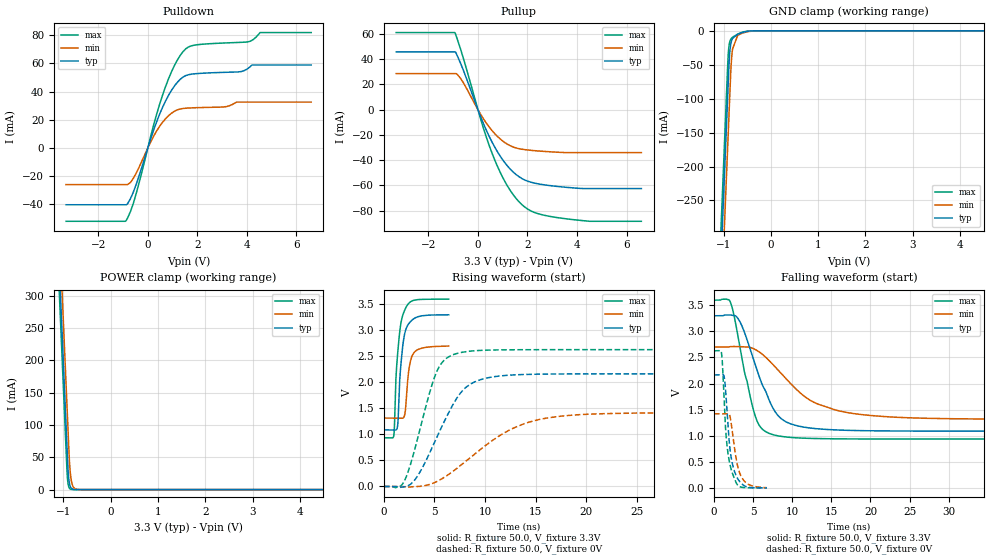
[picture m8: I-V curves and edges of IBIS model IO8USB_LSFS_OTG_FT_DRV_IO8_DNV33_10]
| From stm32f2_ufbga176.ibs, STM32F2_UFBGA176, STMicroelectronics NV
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| *** New cell (Generated with 5.14beta1 (Sep 20 2010 13:23:23))
[Model]   IO8USB_LSFS_OTG_FT_DRV_IO8_DNV33_10
Model_type 3-state
Polarity   Non-Inverting
Enable   Active-Low
| CAP_THRESHOLD on pad DPV33 is "CMOS" :
| Rising=10.0% of vddio   Falling=90.0% of vddio
| C_comp min and max val. don't necessarily correlate with the min and max pvt
| but are the smallest and greatest pad capacitance found.
| var   typ   min   max
C_comp   5.85475pF  5.58530pF  6.39105pF
Vmeas = 1.65V   | Reference voltage for timing measurements
Cref  = 400.0pF   | Timing specification test load capacitance value
Rref  = 1.0MOhm   | Timing specification test load resistance value
Vref  = 1.65V   | Timing specification test load voltage
[Model Spec]
| variable   typ   min   max
[Temperature Range] 25.0 125.0 -40.0
| variable   typ   min   max
[Voltage Range] 3.3V 2.7V 3.6V
| variable   typ   min   max
[POWER Clamp Reference] 3.3V 2.7V 3.6V
| variable   typ   min   max
[GND Clamp Reference] 0V 0V 0V
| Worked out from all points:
|   slope of the pulldown table from 0 to 0.495 V, typ, clamps not added: 20 ohm
|   slope of the pullup table from 0 to 0.495 V, typ, clamps not added: 21.7 ohm
|   GND clamp passes 1 mA (typ) near -0.51 V on its own axis
|   POWER clamp passes 1 mA (typ) near -0.81 V on its own axis
|   rising waveform, R_fixture 50.0, V_fixture 3.3V: 20-80 % time 522ps typ, 458ps min, 538ps max; typ from 1.09 V to 3.3 V
|   falling waveform, R_fixture 50.0, V_fixture 3.3V: 20-80 % time 3.36ns typ, 6.4ns min, 2.22ns max; typ from 3.3 V to 1.09 V
|   rising waveform, R_fixture 50.0, V_fixture 0V: 20-80 % time 3.33ns typ, 6.19ns min, 2.23ns max; typ from 0 V to 2.17 V
|   falling waveform, R_fixture 50.0, V_fixture 0V: 20-80 % time 848ps typ, 986ps min, 769ps max; typ from 2.17 V to 0.001 V
[POWER Clamp]
-3.3V     4.11A      4.173A     4.072A
-1.09V    352.5mA    415.9mA    314.5mA
-1.05V    284.5mA    347.9mA    246.5mA
-1.01V    216.5mA    279.9mA    178.5mA
-920mV    63.51mA    126.9mA    25.85mA
-900mV    31.51mA    92.9mA     9.552mA
-890mV    21.35mA    75.9mA     5.807mA
-870mV    9.804mA    44.01mA    2.146mA
-840mV    3.05mA     18.36mA    482.1uA
-780mV    295.2uA    3.193mA    24.34uA
-660mV    2.775uA    96uA       63.85nA
6.6V      0A         0A         0A
[GND Clamp]
-3.3V     -4.155A    -4.23A     -4.11A
-1.06V    -347.4mA   -421.9mA   -301.9mA
-940mV    -143.4mA   -217.9mA   -97.86mA
-910mV    -92.43mA   -166.9mA   -46.86mA
-890mV    -58.43mA   -132.9mA   -25.36mA
-880mV    -43.4mA    -115.9mA   -20.1mA
-860mV    -25.79mA   -81.93mA   -14.41mA
-840mV    -17.12mA   -51.2mA    -11.69mA
-820mV    -12.64mA   -32.88mA   -10.09mA
-700mV    -5.102mA   -6.6mA     -4.73mA
-230mV    -826nA     -13.68uA   -47.8nA
6.6V      45.45nA    5.674uA    302.2pA
| variable   typ   min   max
[Pullup Reference] 3.3V 2.7V 3.6V
| variable   typ   min   max
[Pulldown Reference] 0V 0V 0V
[Pullup]
-3.3V     45.78mA    28.54mA    61.09mA
-930mV    45.78mA    28.54mA    61.09mA
-700mV    36.69mA    24.76mA    47.9mA
120mV     -6.142mA   -4.065mA   -8.189mA
590mV     -26.5mA    -17.07mA   -35.52mA
1.18V     -44.36mA   -27.27mA   -60.11mA
1.54V     -51.43mA   -30.39mA   -70.35mA
1.89V     -55.75mA   -31.69mA   -77.18mA
2.48V     -58.98mA   -32.83mA   -82.75mA
3.6V      -61.62mA   -34.07mA   -86.61mA
4.51V     -62.54mA   -34.07mA   -88.51mA
6.6V      -62.54mA   -34.07mA   -88.51mA
[Pulldown]
-3.3V     -40.26mA   -25.94mA   -51.99mA
-870mV    -40.25mA   -25.94mA   -51.33mA
-700mV    -35.92mA   -24.51mA   -45.06mA
-470mV    -25.89mA   -17.87mA   -32.39mA
240mV     12.97mA    8.52mA     16.62mA
590mV     28.62mA    18.11mA    37.2mA
1.07V     43.85mA    26mA       58.31mA
1.54V     51.42mA    28.24mA    70.48mA
2.01V     52.82mA    28.63mA    73.27mA
4.01V     56.01mA    32.56mA    75.18mA
4.53V     58.89mA    32.56mA    81.88mA
6.6V      58.89mA    32.56mA    81.88mA
[Ramp]
dV/dt_r 1.29886V/3.33719ns 851.30564mV/6.18971ns 1.57727V/2.2294ns
dV/dt_f 1.32782V/3.35516ns 831.60082mV/6.40782ns 1.59819V/2.21553ns
R_load = 50.0
| Removed startup time: 0s 0s 0s  .
| Removed end time: 6.407ns.
[Rising Waveform]
R_fixture   = 50.0
V_fixture   = 3.3V
V_fixture_min = 2.7V
V_fixture_max = 3.6V
0s        1.087V     1.314V     936.3mV
979ps     1.087V     1.314V     984mV
1.039ns   1.086V     1.314V     1.154V
1.165ns   1.084V     1.314V     1.992V
1.321ns   1.131V     1.314V     2.475V
1.648ns   2.276V     1.313V     3.102V
2.133ns   2.994V     1.483V     3.421V
2.481ns   3.135V     2.262V     3.525V
2.942ns   3.221V     2.562V     3.576V
6.409ns   3.298V     2.697V     3.599V
| Removed startup time: 0s 0s 0s  .
| Removed end time: 44.145ns.
[Falling Waveform]
R_fixture   = 50.0
V_fixture   = 3.3V
V_fixture_min = 2.7V
V_fixture_max = 3.6V
0s        3.3V       2.7V       3.6V
2.1ns     3.314V     2.709V     3.555V
3.385ns   3.163V     2.707V     2.632V
5.16ns    2.412V     2.661V     1.427V
5.915ns   2.074V     2.592V     1.168V
7.115ns   1.657V     2.429V     1.041V
9.56ns    1.241V     2.036V     970.5mV
12.44ns   1.145V     1.667V     948.3mV
16.6ns    1.105V     1.456V     939.3mV
44.16ns   1.087V     1.315V     936.3mV
| Removed startup time: 0s 0s 0s  .
| Removed end time: 35.255ns.
[Rising Waveform]
R_fixture   = 50.0
V_fixture   = 0V
V_fixture_min = 0V
V_fixture_max = 0V
0s        17.03nV    1.21uV     10.92nV
1.995ns   -6.593mV   -4.856mV   96.57mV
3.25ns    179.9mV    -2.259mV   862.3mV
5.1ns     888.7mV    82.89mV    2.15V
5.845ns   1.2V       160.8mV    2.402V
6.88ns    1.591V     298.4mV    2.535V
9.335ns   2.038V     679.2mV    2.612V
12.3ns    2.137V     1.072V     2.626V
15.3ns    2.157V     1.285V     2.628V
35.27ns   2.165V     1.419V     2.629V
| Removed startup time: 0s 0s 0s  .
| Removed end time: 6.76ns.
[Falling Waveform]
R_fixture   = 50.0
V_fixture   = 0V
V_fixture_min = 0V
V_fixture_max = 0V
0s        2.165V     1.419V     2.629V
928ps     2.165V     1.419V     2.603V
1.062ns   2.168V     1.419V     2.399V
1.29ns    2.129V     1.418V     1.665V
1.701ns   1.358V     1.423V     752.4mV
2.033ns   746.8mV    1.371V     447.7mV
2.458ns   391.2mV    927.2mV    235.7mV
3.034ns   174mV      404.2mV    50.77mV
3.672ns   60.28mV    166.7mV    7.902mV
6.762ns   674.8uV    3.311mV    457.1uV
